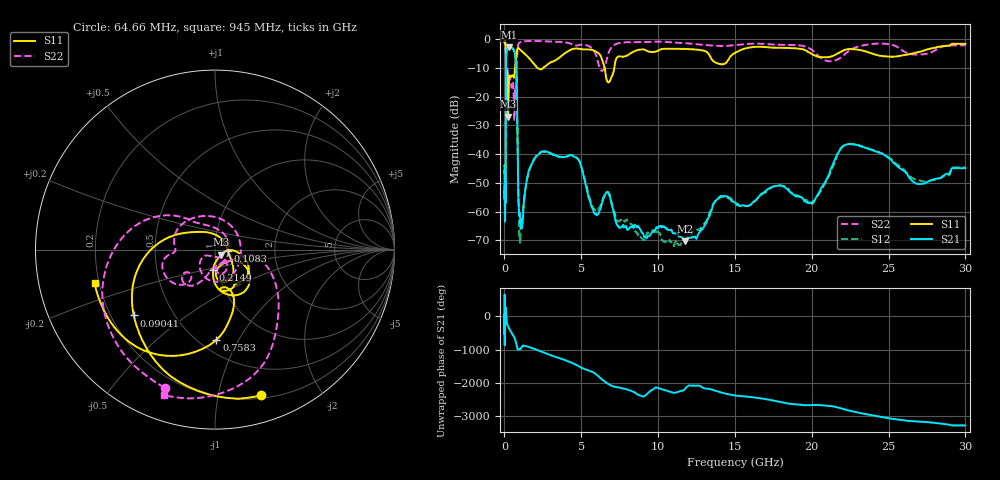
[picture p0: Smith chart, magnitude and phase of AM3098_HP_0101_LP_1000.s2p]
! Date/Time: Thu, Feb 28, 2019 8:36 AM
! Network Analyzer: Agilent Technologies E8364B Rev: A.07.50.67
! Sweep from 0.010 to 30.000 GHz, 1601 Points, Sweep Type: LOG
! Power Supply: 5.022 V, 0.002 A
# Hz S DB R 50
!freq MagS11 AngS11 MagS21 AngS21 MagS12 AngS12 MagS22 AngS22
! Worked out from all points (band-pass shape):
!   1601 points, 10 MHz to 30 GHz, reference 50 ohm
!   highest |S21| = -2.75 dB at 296 MHz (marker M1); lowest = -70.4 dB at 11.77 GHz (marker M2)
!   |S21| within 3 dB of the highest: 114.3 MHz to 706.1 MHz (591.8 MHz wide, 144 % of centre)
!   lowest |S11| = -26.9 dB at 238.7 MHz (marker M3), VSWR 1.09, Z = 53.5 - j3.12 ohm
!   |S11| at or under -10 dB: 97.45 MHz to 682.8 MHz (585.4 MHz wide, 150 % of centre); 2.159 GHz to 2.515 GHz (355.7 MHz wide, 15.2 % of centre); 6.526 GHz to 7.146 GHz (620.3 MHz wide, 9.07 % of centre)
!   |S22| runs from -28.1 to -0.5 dB; largest |S21 - S12| = 0.011
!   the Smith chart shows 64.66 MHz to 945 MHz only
!   S11 on the Smith chart (normalised r, x): 64.66 MHz: 0.23, -1.34; 90.41 MHz: 0.29, -0.33; 108.3 MHz: 1.16, -0.02; 214.9 MHz: 0.95, -0.22; 758.3 MHz: 0.61, -0.81; 945 MHz: 0.18, -0.13
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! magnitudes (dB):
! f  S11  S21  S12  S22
! 10 MHz  -0.4  -46.3  -44.7  -0.6
! 38.04 MHz  -0.5  -61.3  -60.5  -0.9
! 64.66 MHz  -1.4  -52.4  -51.1  -1.7
! 75.13 MHz  -1.9  -52.9  -56.2  -2.3
! 90.41 MHz  -4.7  -32.3  -32.2  -5.2
! 108.3 MHz  -22.7  -7.2  -7.2  -16.2
! 144.7 MHz  -17.8  -3.6  -3.6  -13.8
! 214.9 MHz  -18.8  -3.0  -2.9  -11.7
! 238.7 MHz  -26.9  -2.8  -2.8  -12.7
! 296 MHz  -14.6  -2.7  -2.7  -12.7
! 550.5 MHz  -12.7  -3.4  -3.4  -15.0
! 639.6 MHz  -12.7  -4.1  -4.0  -28.1
! 758.3 MHz  -6.0  -9.1  -9.0  -18.8
! 945 MHz  -3.1  -60.5  -58.6  -1.3
! 1.132 GHz  -4.1  -65.4  -64.7  -0.8
! 2.084 GHz  -9.6  -40.7  -40.6  -0.6
! 4.64 GHz  -3.2  -41.1  -41.1  -2.1
! 7.926 GHz  -5.8  -65.1  -63.0  -1.0
! 11.77 GHz  -3.3  -70.4  -70.2  -1.3
! 20 GHz  -5.1  -56.8  -57.4  -3.6
! 22.56 GHz  -3.4  -36.4  -36.6  -3.5
! 30 GHz  -1.5  -44.9  -44.6  -2.1
